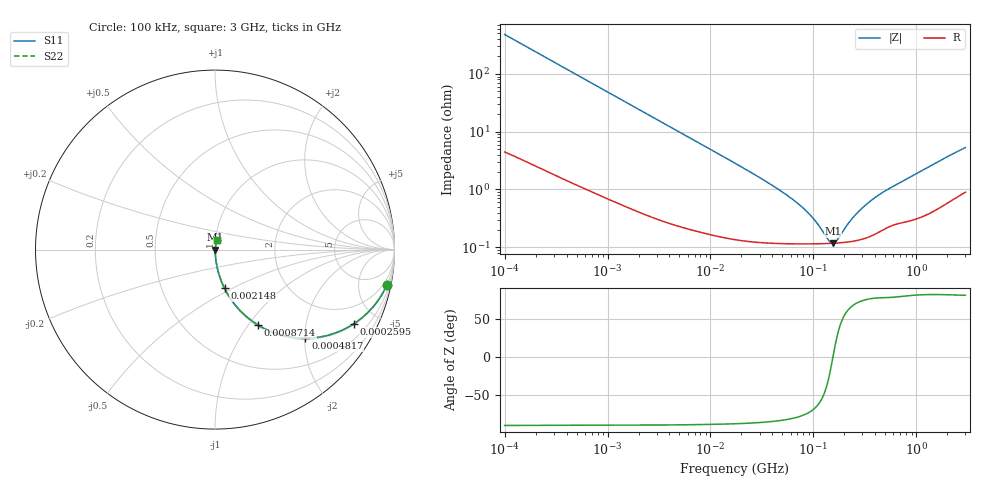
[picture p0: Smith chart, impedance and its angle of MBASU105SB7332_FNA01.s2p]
! MBASU105SB7332_FNA01  S-PARAMETER MODEL  ( Standard Model )
! Model Generated by TAIYO YUDEN Corporation (http://www.ty-top.com)
! Version 1.0
! TAIYO YUDEN Control No. 220601
! Copyright(c) 2013 TAIYO YUDEN CO.,LTD. All Rights Reserved.
! Product Description (link to TY-COMPAS)
! https://ds.yuden.co.jp/TYCOMPAS/or/detail?pn=MBASU105SB7332KFNA01&u=M
! Products Name : Multilayer Ceramic Capacitors
! Characteristics :
!  Capacitance : 3300 [pF] , Rated Voltage : 50 [V] , TCC : X7R
!  Case Size : 1.0 x 0.5 / 0.039 x 0.02 [mm/inch] , Thickness : 0.5 / 0.02 [mm/inch]
!  (Conditions: Temperature = 25 [degC] , DC Bias Voltage = 0 [V])
! External Node Assignments :
!  1  o---| |---o  2
! GND o---------o GND
! Frequency Range : 100kHz  -  3GHz  [ 401 STEP ]
# MHZ S RI R 50
! Freq[MHz].  S11 Real  S11 Imag  S21 Real  S21 Imag  S12 Real  S12 Imag  S22 Real  S22 Imag
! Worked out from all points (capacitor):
!   401 points, 100 kHz to 3 GHz, reference 50 ohm
!   read as one part in series: C = 3.31 nF near 105.3 kHz
!   lowest |Z| = 118 mohm at 154.9 MHz (marker M1)
!   series resonance near 155 MHz, so ESL is about 320 pH
!   S11 on the Smith chart (normalised r, x): 100 kHz: 1.09, -9.60; 259.5 kHz: 1.04, -3.72; 481.7 kHz: 1.02, -2.01; 871.4 kHz: 1.02, -1.12; 2.148 MHz: 1.01, -0.46; 3 GHz: 1.02, +0.10
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0.1  0.9567 -0.1989  0.0433 0.1989  0.0433 0.1989  0.9567 -0.1989
0.167439  0.8897 -0.3082  0.1103 0.3082  0.1103 0.3082  0.8897 -0.3082
0.259498  0.7735 -0.4131  0.2265 0.4131  0.2265 0.4131  0.7735 -0.4131
0.481683  0.5035 -0.4939  0.4965 0.4939  0.4965 0.4939  0.5035 -0.4939
0.562235  0.4282 -0.4886  0.5718 0.4886  0.5718 0.4886  0.4282 -0.4886
0.871356  0.2413 -0.421  0.7587 0.421  0.7587 0.421  0.2413 -0.421
1.316074  0.1249 -0.3232  0.8751 0.3232  0.8751 0.3232  0.1249 -0.3232
2.147551  0.0529 -0.2156  0.9471 0.2156  0.9471 0.2156  0.0529 -0.2156
3.161081  0.0264 -0.1511  0.9736 0.1511  0.9736 0.1511  0.0264 -0.1511
6.674626  0.0074 -0.0734  0.9926 0.0734  0.9926 0.0734  0.0074 -0.0734
17.7727  0.00211 -0.0276  0.9979 0.0276  0.9979 0.0276  0.00211 -0.0276
53.83243  0.00122 -0.00817  0.9988 0.00817  0.9988 0.00817  0.00122 -0.00817
75.25761  0.00117 -0.00508  0.9988 0.00508  0.9988 0.00508  0.00117 -0.00508
97.38194  0.00116 -0.00311  0.9988 0.00311  0.9988 0.00311  0.00116 -0.00311
139.694  0.00116 -0.000674  0.9988 0.000674  0.9988 0.000674  0.00116 -0.000674
154.8634  0.00117 -5.69e-06  0.9988 5.69e-06  0.9988 5.69e-06  0.00117 -5.69e-06
171.6802  0.00119 0.000663  0.9988 -0.000663  0.9988 -0.000663  0.00119 0.000663
227.9507  0.00126 0.00257  0.9987 -0.00257  0.9987 -0.00257  0.00126 0.00257
287.4592  0.00137 0.00427  0.9986 -0.00427  0.9986 -0.00427  0.00137 0.00427
391.6425  0.00171 0.00689  0.9983 -0.00689  0.9983 -0.00689  0.00171 0.00689
547.5153  0.00237 0.0101  0.9976 -0.0101  0.9976 -0.0101  0.00237 0.0101
3000  0.0116 0.0513  0.9884 -0.0513  0.9884 -0.0513  0.0116 0.0513
